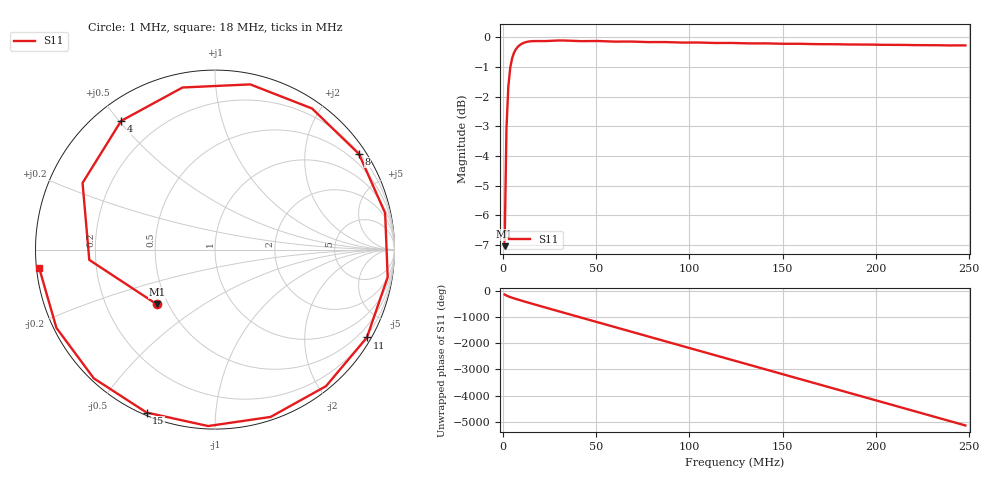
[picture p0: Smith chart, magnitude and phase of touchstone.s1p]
# MHz S RI R 50.0
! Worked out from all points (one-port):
!   248 points, 1 MHz to 248 MHz, reference 50 ohm
!   lowest |S11| = -7.0 dB at 1 MHz (marker M1), VSWR 2.60, Z = 21.7 - j16.5 ohm
!   |S11| at or under -10 dB: nowhere
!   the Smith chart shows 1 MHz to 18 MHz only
!   S11 on the Smith chart (normalised r, x): 1 MHz: 0.43, -0.33; 4 MHz: 0.07, +0.51; 8 MHz: 0.22, +3.30; 11 MHz: 0.17, -3.72; 15 MHz: 0.01, -0.66; 18 MHz: 0.01, -0.05
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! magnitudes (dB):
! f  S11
! 1 MHz  -7.0
! 2 MHz  -3.1
! 3 MHz  -1.7
! 4 MHz  -1.0
! 5 MHz  -0.7
! 6 MHz  -0.5
! 7 MHz  -0.4
! 8 MHz  -0.3
! 9 MHz  -0.3
! 11 MHz  -0.2
! 13 MHz  -0.2
! 15 MHz  -0.1
! 18 MHz  -0.1
! 32 MHz  -0.1
! 40 MHz  -0.1
! 49 MHz  -0.1
! 58 MHz  -0.1
! 63 MHz  -0.1
! 68 MHz  -0.1
! 77 MHz  -0.2
! 86 MHz  -0.2
! 94 MHz  -0.2
! 103 MHz  -0.2
! 125 MHz  -0.2
! 156 MHz  -0.2
! 187 MHz  -0.2
! 218 MHz  -0.3
! 248 MHz  -0.3
